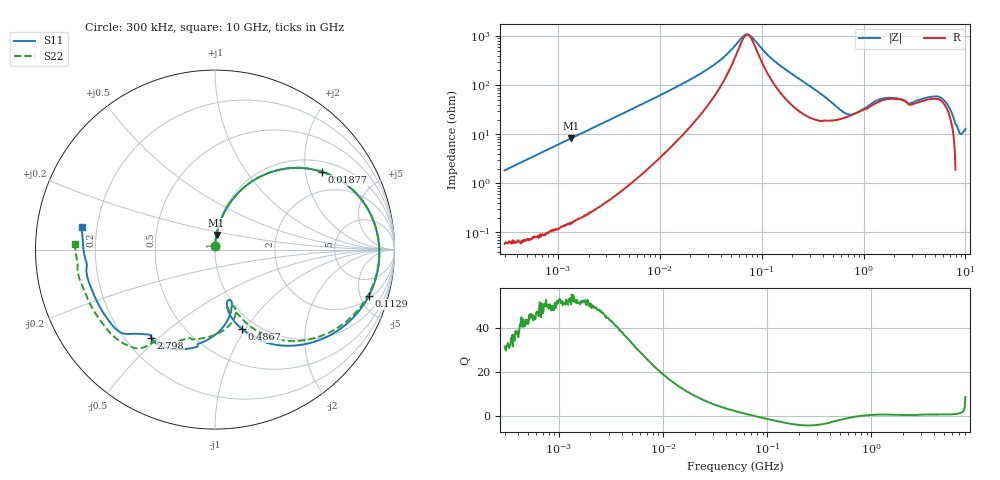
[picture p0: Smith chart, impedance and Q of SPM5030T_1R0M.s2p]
! S-Parameter Data Generated by TDK Corporation
! Copyright(C) 2023 TDK Corporation.
! All Rights Reserved.
! TDK P/N: SPM5030T-1R0M (Inductor)
! Property: L=1uH at 100kHz
! Size(LxWxT): 5.2x5x3mm
! Model Type: s2p (Touchstone File Format Version 1.0)
! Frequency: DC=Yes Start=0.3MHz Stop=10000MHz 802points Log-sweep
! Model Generated on Sep. 29, 2023
! Port Assignments:
!  1 ---@@@--- 2
! Applicable Conditions:
!  Temperature = 25 degC
!  DC Bias Current = 0 A
!  Small Signal Operation
! Terms and conditions regarding TDK Simulation Models
! (1)This simulation model is being provided solely for informational purposes. Please refer to the specifications of the products in terms of detailed characteristics of such products.
! (2)In no event shall TDK Corporation of any of its subsidiaries be liable for any loss or damage arising, directly or indirectly,
!  From any information contained in this simulation model, including, but not limited to loss or damages arising from any inaccuracies, omissions or errors in connection with such information.
! (3)Any and all copyrights on this simulation model are owned by TDK Corporation.
!  Duplication or redistribution of this simulation model without prior written permission from TDK Corporation is prohibited.
! (4)This simulation model is subject to any modification or change without any prior notice.
! (5)Neither TDK Corporation nor any of its subsidiaries shall make any warranty, express or implied,
!  Including but not limited to the correctness, implied warranties of merchantability and fitness for a particular purpose with respect to this simulation models.
! (6)The use of this simulation model shall be deemed to have consented to the terms and conditions hereof.
# Hz S MA R 50
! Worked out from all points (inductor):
!   801 points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, 300 kHz to 10 GHz, reference 50 ohm
!   read as one part in series: L = 976 nH near 318.3 kHz
!   highest Q = 52.8 at 1.356 MHz (marker M1), where L = 976 nH
!   self-resonance near 72.4 MHz
!   S11 on the Smith chart (normalised r, x): 300 kHz: 1.00, +0.04; 18.77 MHz: 1.30, +2.46; 112.9 MHz: 2.30, -5.94; 486.7 MHz: 0.85, -0.97; 2.798 GHz: 0.30, -0.47; 10 GHz: 0.14, +0.08
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300000  0.01804 87.2  0.9993 -1.1  0.9992 -1.1  0.01796 86.9
1355528  0.08222 84.1  0.9951 -4.8  0.995 -4.8  0.0822 84.1
1713600  0.1035 82.9  0.9926 -6.0  0.9927 -6.0  0.1036 82.9
4734969  0.2748 72.1  0.9535 -16.2  0.9534 -16.2  0.2748 72.2
9671944  0.5004 56.6  0.8402 -30.4  0.8403 -30.4  0.5003 56.7
1.877128e7  0.7356 36.1  0.6063 -47.9  0.6063 -47.9  0.7354 36.3
3.467969e7  0.8722 16.8  0.3274 -59.6  0.3274 -59.6  0.8718 17.2
5.477226e7  0.9115 3.8  0.1425 -50.7  0.1425 -50.7  0.9109 4.5
7.329659e7  0.916 -4.1  0.08456 -0.1  0.08459 -0.1  0.9152 -3.3
1.128912e8  0.8951 -16.7  0.2066 48.9  0.2067 48.9  0.8942 -15.3
2.013356e8  0.7972 -36.9  0.4541 41.8  0.4541 41.8  0.7977 -34.3
3.126428e8  0.6537 -54.9  0.6314 25.5  0.6315 25.5  0.6585 -50.7
4.866838e8  0.469 -71.1  0.7386 5.0  0.7386 5.0  0.4886 -64.2
9.445544e8  0.2909 -74.7  0.7001 -29.4  0.7002 -29.4  0.3572 -75.8
1.292013e9  0.354 -75.4  0.6238 -46.2  0.6238 -46.2  0.3996 -74.6
1.767019e9  0.4832 -91.3  0.4971 -60.3  0.4971 -60.3  0.493 -96.0
2.264206e9  0.5882 -109.1  0.4221 -69.2  0.4221 -69.2  0.5412 -110.8
2.798208e9  0.6057 -125.9  0.4039 -76.9  0.4039 -76.9  0.6003 -121.3
5.526371e9  0.7075 -141.4  0.1966 -116.3  0.1966 -116.4  0.7387 -137.4
6.737565e9  0.7162 -152.7  0.1715 -128.1  0.1715 -128.1  0.7549 -151.8
8.881947e9  0.7334 179.6  0.1258 -150.4  0.1258 -150.4  0.7789 179.1
1e10  0.7508 170.3  0.1031 -157.0  0.1031 -157.0  0.7827 177.7
